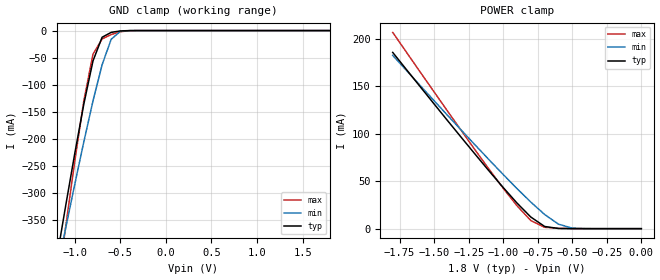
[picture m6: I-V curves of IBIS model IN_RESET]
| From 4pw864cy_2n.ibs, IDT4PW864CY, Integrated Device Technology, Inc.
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|   Model IN_RESET
[Model]   IN_RESET
Model_type   Input
Vinl =  0.59500V
Vinh =  1.23500V
C_comp   1.750000pF   1.75000pF   1.75000pF
[Temperature Range]   25.00000   0.11000k   0.000
[Voltage Range]   1.80000V   1.70000V   1.90000V
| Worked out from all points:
|   GND clamp passes 1 mA (typ) near -0.51 V on its own axis
|   POWER clamp passes 1 mA (typ) near -0.64 V on its own axis
[GND_clamp]
| voltage   I(typ)   I(min)   I(max)
-1.8V     -1.042A    -958.3mA   -1.272A
-1.2V     -424.1mA   -448.5mA   -489.1mA
-1.1V     -324.5mA   -365.8mA   -363.4mA
-1V       -227.5mA   -284.5mA   -241.9mA
-900mV    -135.5mA   -205.4mA   -129.3mA
-800mV    -56.14mA   -130.2mA   -43.72mA
-700mV    -12.34mA   -63.12mA   -15.49mA
-600mV    -3.312mA   -15.96mA   -7.316mA
-500mV    -636.5uA   -1.447mA   -2.163mA
-300mV    -2.084uA   -3.939uA   -9.999uA
1.8V      25.37pA    8.201nA    -20.58pA
[POWER_clamp]
| voltage   I(typ)   I(min)   I(max)
-1.8V     185.8mA    182.7mA    206.9mA
-1.4V     113.4mA    119mA      123.3mA
-1.1V     60.42mA    72.28mA    62.15mA
-900mV    26.99mA    42.23mA    24.11mA
-800mV    12.24mA    27.99mA    8.537mA
-700mV    2.309mA    14.93mA    1.433mA
-600mV    187.3uA    4.737mA    363.9uA
-500mV    22.39uA    519.1uA    71.04uA
0V        25.37pA    590pA      7.891pA
